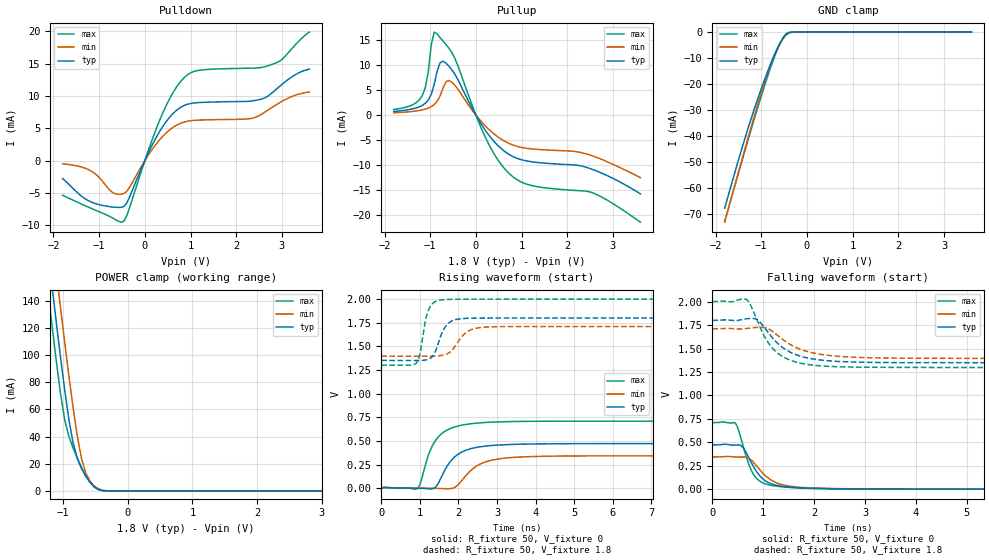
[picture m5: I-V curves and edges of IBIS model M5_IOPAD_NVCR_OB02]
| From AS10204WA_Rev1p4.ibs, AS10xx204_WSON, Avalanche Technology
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[Model] M5_IOPAD_NVCR_OB02
Model_type I/O
Enable   Active-High
Vinl  =  0.54
Vinh  =  1.26
Vmeas =  0.9
Cref  =  30e-12
| Capacitance  typ   min   max
C_comp   3.869840e-12   3.575244e-12   4.208825e-12
| Variables   typ   min   max
[GND Clamp Reference]   0   0   0
[POWER Clamp Reference]   1.8   1.71   2
[Pulldown Reference]   0   0   0
[Pullup Reference]   1.8   1.71   2
[Temperature Range]   25   105   -40
[Voltage Range]   1.8   1.71   2
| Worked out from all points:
|   slope of the pulldown table from 0 to 0.27 V, typ, clamps not added: 70.1 ohm
|   slope of the pullup table from 0 to 0.27 V, typ, clamps not added: 70.5 ohm
|   GND clamp passes 1 mA (typ) near -0.46 V on its own axis
|   POWER clamp passes 1 mA (typ) near -0.44 V on its own axis
|   falling waveform, R_fixture 50, V_fixture 0: 20-80 % time 352ps typ, 430ps min, 280ps max; typ from 0.471 V to 0 V
|   falling waveform, R_fixture 50, V_fixture 1.8: 20-80 % time 579ps typ, 679ps min, 480ps max; typ from 1.8 V to 1.35 V
|   rising waveform, R_fixture 50, V_fixture 0: 20-80 % time 529ps typ, 611ps min, 463ps max; typ from 0 V to 0.471 V
|   rising waveform, R_fixture 50, V_fixture 1.8: 20-80 % time 269ps typ, 371ps min, 192ps max; typ from 1.35 V to 1.8 V
[GND Clamp]
| Voltage   I(typ)   I(min)   I(max)
-1.8V     -67.84mA   -73.19mA   -72.81mA
-1.499V   -49.26mA   -53.93mA   -54.28mA
-1.303V   -37.87mA   -41.64mA   -42.4mA
-1.108V   -27.29mA   -29.68mA   -30.84mA
-912.4mV  -17.6mA    -18.46mA   -19.84mA
-782.1mV  -11.7mA    -11.87mA   -13.01mA
-651.7mV  -6.447mA   -6.494mA   -6.896mA
-521.4mV  -2.255mA   -2.526mA   -2.141mA
-456.2mV  -849.3uA   -1.156mA   -679.4uA
-391mV    -172uA     -356.5uA   -88.88uA
-260.7mV  -2.088uA   -12.98uA   -254.3nA
3.6V      0A         0A         0A
[POWER Clamp]
| Voltage   I(typ)   I(min)   I(max)
-1.8V     419.8mA    456.6mA    390.9mA
-1.238V   178mA      215.7mA    148.4mA
-1.173V   151mA      188.6mA    121.7mA
-1.108V   124.5mA    161.8mA    96mA
-1.043V   98.85mA    135.4mA    72.14mA
-977.6mV  74.56mA    109.6mA    52.56mA
-912.4mV  52.76mA    84.78mA    40.16mA
-847.2mV  35.48mA    61.36mA    31.71mA
-716.9mV  16.42mA    23.91mA    17.31mA
-651.7mV  10.9mA     13.27mA    11.28mA
-456.2mV  1.168mA    1.554mA    921.1uA
3.6V      0A         0A         0A
[Pulldown]
| Voltage   I(typ)   I(min)   I(max)
-1.8V     -2.779mA   -490.2uA   -5.361mA
-1.173V   -6.412mA   -1.619mA   -7.394mA
-716.9mV  -7.17mA    -4.875mA   -8.838mA
-456.2mV  -7.098mA   -5.081mA   -9.361mA
310.3mV   4.353mA    3.118mA    6.008mA
620.7mV   7.316mA    5.162mA    10.57mA
869mV     8.567mA    5.992mA    12.9mA
1.241V    9.008mA    6.289mA    14.03mA
2.352V    9.244mA    6.558mA    14.31mA
2.766V    10.37mA    8.15mA     14.85mA
2.972V    11.63mA    9.056mA    15.49mA
3.6V      14.16mA    10.62mA    19.89mA
[Pullup]
| Voltage   I(typ)   I(min)   I(max)
-1.8V     713.6uA    450.5uA    1.098mA
-1.173V   1.921mA    1.031mA    3.898mA
-1.043V   2.99mA     1.386mA    8.588mA
-977.6mV  4.11mA     1.67mA     14mA
-912.4mV  6.104mA    2.089mA    16.54mA
-782.1mV  10.46mA    3.84mA     15.4mA
-651.7mV  10.31mA    6.664mA    14.04mA
-456.2mV  8.081mA    5.895mA    11.23mA
248.3mV   -3.569mA   -2.543mA   -5.217mA
744.8mV   -7.943mA   -5.724mA   -11.78mA
2.559V    -10.86mA   -8.148mA   -15.51mA
3.6V      -15.7mA    -12.46mA   -21.35mA
[Ramp]
dV/dt_r   0.282807/0.529465n  0.205561/0.611231n  0.425437/0.462933n
dV/dt_f   0.271206/0.579502n  0.189603/0.679401n  0.421848/0.479962n
R_load = 50
[Falling Waveform]
R_fixture = 50
V_fixture = 0
V_fixture_min = 0
V_fixture_max = 0
| Time   V(typ)   V(min)   V(max)
0s        471.3mV    342.6mV    709.1mV
456.1ps   470mV      342.1mV    699.6mV
507.4ps   472.5mV    342.4mV    640.9mV
592.1ps   450.1mV    343.8mV    482.5mV
743.8ps   304.7mV    319.4mV    226.6mV
918.2ps   151.1mV    215.7mV    90.72mV
1.181ns   52.65mV    88.37mV    38.3mV
1.537ns   20.7mV     30.35mV    17.55mV
3.803ns   825.3uV    737.2uV    443.9uV
21.88ns   148.3nV    492.5nV    196.1nV
[Falling Waveform]
R_fixture = 50
V_fixture = 1.8
V_fixture_min = 1.71
V_fixture_max = 2
| Time   V(typ)   V(min)   V(max)
0s        1.8V       1.71V      2V
668.7ps   1.817V     1.714V     2.023V
757.8ps   1.82V      1.72V      1.955V
896ps     1.802V     1.725V     1.779V
1.076ns   1.686V     1.717V     1.579V
1.279ns   1.556V     1.64V      1.452V
1.683ns   1.426V     1.502V     1.35V
2.237ns   1.371V     1.429V     1.311V
4.028ns   1.349V     1.396V     1.298V
21.88ns   1.348V     1.394V     1.297V
[Rising Waveform]
R_fixture = 50
V_fixture = 0
V_fixture_min = 0
V_fixture_max = 0
| Time   V(typ)   V(min)   V(max)
0s        64.51nV    381.8nV    117.5nV
929.7ps   137.8uV    895.5uV    -4.858mV
1.021ns   -1.205mV   818.9uV    63.07mV
1.241ns   -8.135mV   -190.2uV   372.4mV
1.458ns   37.82mV    -2.201mV   533.9mV
1.889ns   326.4mV    5.748mV    645.9mV
2.545ns   436.5mV    251.1mV    690.7mV
3.173ns   459.1mV    316.6mV    702.8mV
4.495ns   469.7mV    339mV      708.3mV
21.88ns   471.3mV    342.6mV    709.1mV
[Rising Waveform]
R_fixture = 50
V_fixture = 1.8
V_fixture_min = 1.71
V_fixture_max = 2
| Time   V(typ)   V(min)   V(max)
0s        1.348V     1.394V     1.297V
908.2ps   1.349V     1.395V     1.323V
987.9ps   1.35V      1.395V     1.397V
1.13ns    1.354V     1.395V     1.742V
1.237ns   1.366V     1.395V     1.897V
1.37ns    1.419V     1.396V     1.966V
1.649ns   1.701V     1.412V     1.995V
2.252ns   1.797V     1.661V     1.999V
2.872ns   1.799V     1.707V     1.999V
21.88ns   1.8V       1.71V      2V
